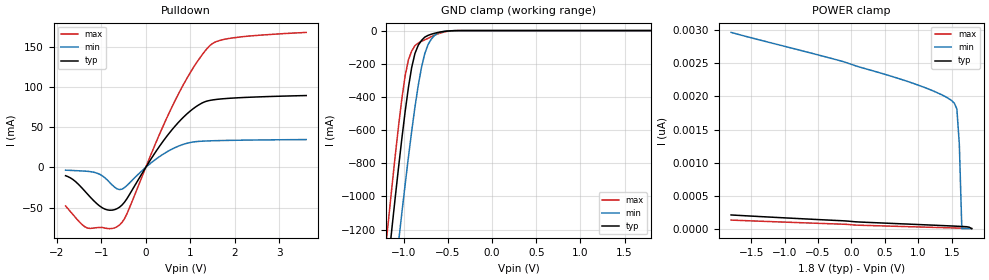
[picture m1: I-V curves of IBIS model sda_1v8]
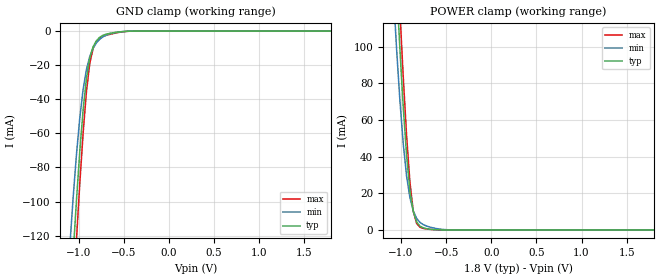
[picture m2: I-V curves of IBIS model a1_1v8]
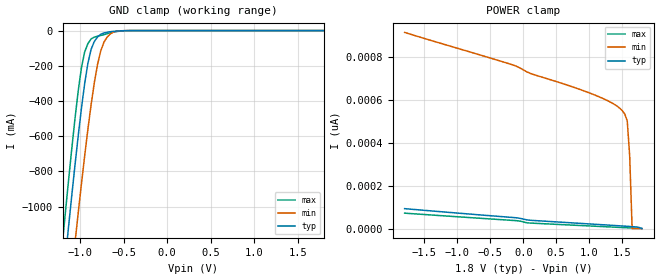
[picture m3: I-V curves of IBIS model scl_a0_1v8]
| Texas Instruments Incorporated
| Marketing Part # : ADS112C14, ADS122C14
| Digital Voltage Range : 1.65V - 3.6V
| Package-type: QFN-RTE
| #pins/pkg drawing : QFN-16
[IBIS ver] 7.0
[File name]  ads112c14_ads122c14.ibs
[File Rev]  1.0
[Date]   08 10, 2026
[Source]
| Texas Instruments Incorporated.
| 12500 TI Blvd
| Dallas, TX -75243
[Notes] Revision History:
| Rev 1.0: 08/10/2026
| - Initial version of the model
| - Model generated from simulations in TISPICE/SPECTRE
| - C_comp although listed in numerical order of value are
|   obtained from varying PVT conditions. For PVT conditions for
|   each specific value refer the buffer description under
|   respective [Model]. IBIS model user is responsible for using
|   appropriate C_comp to simulate for Signal Integrity.
| - Warnings regarding combined Non-monotonicity of various models have been
| reviewed and considered minor and can be ignored.
| - Model names with a trailing _1v8 contain the model for 1.8V operation.
| - Model names with a trailing _3v3 contain the model for 3.3V operation.
[Disclaimer]
| This model is designed as an aid for customers of Texas Instruments.
| TI and its licensors and suppliers make no warranties, either expressed
| or implied, with respect to this model, including the warranties of
| merchantability or fitness for a particular purpose. The model is
| provided solely on an "as is" basis. The entire risk as to its quality
| and performance is with the customer.
| This model is subject to change without notice. Texas Instruments
| Incorporated is not responsible for updating this model.
[Copyright]
(C) Copyright 2026 Texas Instruments Incorporated. All rights reserved.
| Component1 ADS1x2C14RTE
[Component] ADS1x2C14RTE
[Manufacturer] Texas Instruments Incorporated
[Package] |16 WQFN - RUK package
| variable   typ   min   max
R_pkg   50.000m   25.000m   100.000m
L_pkg   0.500nH   0.250nH   1.000nH
C_pkg   0.100pF   50.000fF   0.200pF
| pin number (pin name) mapping to model name
[Pin] signal_name   model_name   R_pin   L_pin   C_pin
1   AIN0   NC   NA   NA   NA
2   AIN1   NC   NA   NA   NA
3   AIN2   NC   NA   NA   NA
4   AIN3   NC   NA   NA   NA
5   AIN4   NC   NA   NA   NA
6   AIN5   NC   NA   NA   NA
7   AIN6   NC   NA   NA   NA
8   AIN7   NC   NA   NA   NA
9   A0   input_scl_a0   NA   NA   NA
10   A1   input_a1   NA   NA   NA
11   SDA   inout_sda   NA   NA   NA
12   SCL   input_scl_a0   NA   NA   NA
13   IOVDD   NC   NA   NA   NA
14   GND   NC   NA   NA   NA
15   AVDD   NC   NA   NA   NA
16   REFOUT   NC   NA   NA   NA
|***** end of component 1 definition
|***** Model Selections ********
|***** Power supply options *********
[Model Selector] input_scl_a0
scl_a0_1v8 input buffer at 1.8V operation.
scl_a0_3v3 input buffer at 3.3V operation.
[Model Selector] input_a1
a1_1v8 input buffer at 1.8V operation.
a1_3v3 input buffer at 3.3V operation.
[Model Selector] inout_sda
sda_1v8 input buffer at 1.8V operation.
sda_3v3 input buffer at 3.3V operation.
| Models and submodels in the file (6): sda_1v8 (I/O_open_drain), a1_1v8 (Input), scl_a0_1v8 (Input), sda_3v3 (I/O_open_drain), a1_3v3 (Input), scl_a0_3v3 (Input)
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|   Model sda_1v8
[Model] sda_1v8
Model_type I/O_open_drain
Polarity   Non-Inverting
Enable   Active-High
Vinl =  0.540V
Vinh =  1.260V
C_comp   4.000pF   2.000pF   8.000pF
[Model Spec]
Vinh   1.260V   1.115V   1.365V
Vinl   0.540V   0.494V   0.585V
[Temperature Range]   27.000   0.125k   -40.000
[Voltage Range]   1.800V   1.650V   1.950V
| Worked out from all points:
|   slope of the pulldown table from 0 to 0.27 V, typ, clamps not added: 11.6 ohm
|   GND clamp passes 1 mA (typ) near -0.45 V on its own axis
[Pulldown]
|Voltage   I(typ)   I(min)   I(max)
-1.8V     -10.4mA    -3.493mA   -48.03mA
-1.305V   -33.42mA   -4.939mA   -75.58mA
-920mV    -51.9mA    -12.84mA   -75.51mA
-590mV    -49.56mA   -27.68mA   -71.73mA
-425mV    -39.17mA   -22.74mA   -58.04mA
125mV     11.07mA    5.793mA    17.14mA
620mV     48.89mA    23.6mA     78.83mA
1.005V    70.39mA    30.99mA    118.5mA
1.39V     82.68mA    32.88mA    148.7mA
1.555V    84.3mA     33.18mA    155.8mA
1.885V    85.95mA    33.58mA    160.5mA
3.6V      89.34mA    34.58mA    167.9mA
[GND_clamp]
|Voltage   I(typ)   I(min)   I(max)
-1.8V     -4.499A    -4.387A    -4.584A
-1.208V   -1.559A    -1.997A    -1.316A
-1.171V   -1.369A    -1.813A    -1.122A
-1.134V   -1.183A    -1.63A     -932.1mA
-1.06V    -820.7mA   -1.272A    -571mA
-986mV    -488mA     -927.3mA   -271.8mA
-912mV    -222.4mA   -606.8mA   -123.5mA
-838mV    -88.72mA   -331.1mA   -75.13mA
-764mV    -39.58mA   -139.3mA   -55.93mA
-653mV    -16.25mA   -29.74mA   -27.62mA
-505mV    -2.763mA   -2.319mA   -4.524mA
1.8V      0A         0A         0A
[POWER_clamp]
|Voltage   I(typ)   I(min)   I(max)
-1.8V     207.2pA    2.969nA    129.5pA
-161mV    120.8pA    2.538nA    68.73pA
653mV     77.38pA    2.288nA    36.1pA
1.208V    53.49pA    2.09nA     20.03pA
1.393V    45.32pA    2.004nA    14.75pA
1.504V    40.28pA    1.933nA    11.59pA
1.541V    38.55pA    1.895nA    10.54pA
1.578V    36.8pA     1.81nA     9.496pA
1.615V    35.01pA    1.272nA    8.449pA
1.652V    33.18pA    0A         7.403pA
1.763V    21.8pA     0A         4.268pA
1.8V      0A         0A         3.223pA
[Ramp]
| variable   typ   min   max
dV/dt_r   1.068/4.090n   0.970/3.973n   1.162/4.162n
dV/dt_f   1.068/0.405n   0.970/0.745n   1.162/0.243n
R_load = 1.000k
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|   Model a1_1v8
[Model] a1_1v8
Model_type Input
Polarity   Non-Inverting
Enable   Active-High
Vinl =  0.540V
Vinh =  1.260V
C_comp   1.600pF   0.800pF   3.200pF
[Model Spec]
Vinh   1.260V   1.155V   1.365V
Vinl   0.540V   0.495V   0.585V
[Temperature Range]   27.000   0.125k   -40.000
[Voltage Range]   1.800V   1.650V   1.950V
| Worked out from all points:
|   GND clamp passes 1 mA (typ) near -0.62 V on its own axis
|   POWER clamp passes 1 mA (typ) near -0.74 V on its own axis
[GND_clamp]
|Voltage   I(typ)   I(min)   I(max)
-1.8V     -906.9mA   -836.6mA   -952.9mA
-1.097V   -165.1mA   -126.9mA   -194.1mA
-1.06V    -131.4mA   -98.21mA   -157.8mA
-1.023V   -99.65mA   -72.66mA   -122.8mA
-986mV    -70.87mA   -51.1mA    -89.77mA
-949mV    -46.4mA    -34.34mA   -60.03mA
-912mV    -27.77mA   -22.5mA    -35.52mA
-875mV    -15.77mA   -14.85mA   -18.82mA
-838mV    -9.16mA    -10.03mA   -10.16mA
-764mV    -3.557mA   -4.737mA   -4.173mA
-431mV    -56.83uA   -62.45uA   -67.68uA
1.8V      0A         0A         0A
[POWER_clamp]
|Voltage   I(typ)   I(min)   I(max)
-1.8V     957.9mA    899.5mA    993.1mA
-1.086V   170mA      130.8mA    195.3mA
-1.049V   133.3mA    98.81mA    156.6mA
-1.012V   98.55mA    70.47mA    119mA
-975mV    66.97mA    46.97mA    83.44mA
-938mV    40.49mA    29.36mA    51.44mA
-901mV    21.29mA    17.57mA    25.92mA
-864mV    9.938mA    10.42mA    10.21mA
-827mV    4.429mA    6.356mA    3.552mA
-790mV    2.115mA    4.139mA    1.502mA
-457mV    2.391uA    60.32uA    338.6nA
1.8V      0A         0A         0A
|   Model scl_a0_1v8
[Model] scl_a0_1v8
Model_type Input
Polarity   Non-Inverting
Enable   Active-High
Vinl =  0.540V
Vinh =  1.260V
C_comp   1.000pF   0.500pF   2.000pF
[Model Spec]
Vinh   1.260V   1.155V   1.365V
Vinl   0.540V   0.495V   0.585V
[Temperature Range]   27.000   0.125k   -40.000
[Voltage Range]   1.800V   1.650V   1.950V
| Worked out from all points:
|   GND clamp passes 1 mA (typ) near -0.51 V on its own axis
[GND_clamp]
|Voltage   I(typ)   I(min)   I(max)
-1.8V     -4.321A    -4.211A    -4.387A
-1.208V   -1.482A    -1.911A    -1.228A
-1.171V   -1.298A    -1.732A    -1.039A
-1.134V   -1.117A    -1.554A    -853.4mA
-1.06V    -766mA     -1.207A    -501.9mA
-1.023V   -599.9mA   -1.038A    -344.6mA
-949mV    -303.3mA   -714.6mA   -122.5mA
-875mV    -107.5mA   -423.2mA   -47.74mA
-764mV    -20.72mA   -115.9mA   -27.81mA
-690mV    -9.399mA   -36.96mA   -17.74mA
-616mV    -4.409mA   -7.887mA   -8.375mA
1.8V      0A         0A         0A
[POWER_clamp]
|Voltage   I(typ)   I(min)   I(max)
-1.8V     93.02pA    912.5pA    72.11pA
-124mV    51.09pA    757.6pA    37.67pA
135mV     38.47pA    718.9pA    25.58pA
764mV     26.5pA     657.5pA    16.14pA
1.134V    19.53pA    615.2pA    10.66pA
1.356V    15.29pA    582.7pA    7.391pA
1.467V    13.13pA    559.2pA    5.763pA
1.541V    11.65pA    532.4pA    4.678pA
1.578V    10.89pA    500.5pA    4.137pA
1.615V    10.12pA    337.4pA    3.595pA
1.652V    9.318pA    0A         3.054pA
1.8V      0A         0A         888.5fA
